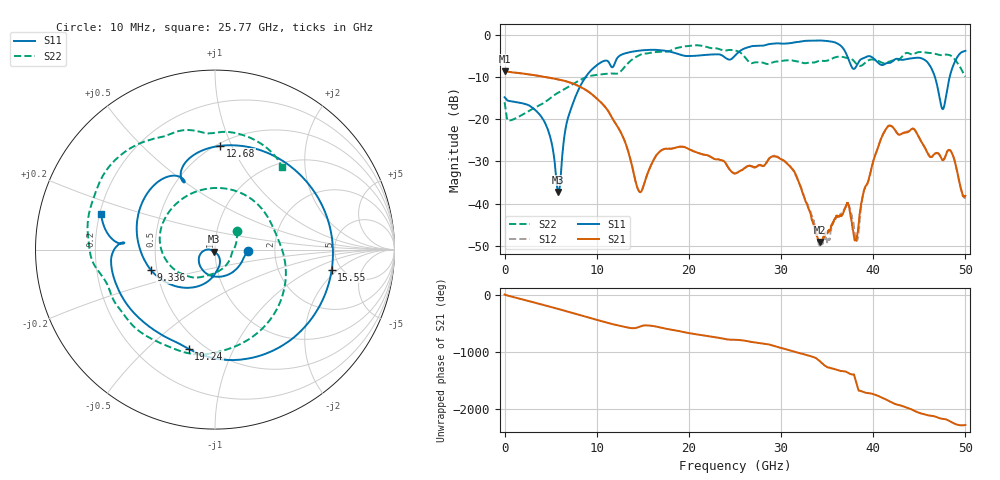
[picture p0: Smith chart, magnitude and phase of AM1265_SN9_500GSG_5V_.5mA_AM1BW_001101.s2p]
!Keysight Technologies,N5245B,MY58422270,A.16.20.02
!Date: Thursday, March 05, 2026 00:44:23
!Correction: S11(C  2-Port  )
!S21(C  2-Port  )
!S12(C  2-Port  )
!S22(C  2-Port  )
!S2P File: Measurements: S11, S21, S12, S22:
# Hz S  dB  R 50
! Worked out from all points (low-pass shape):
!   3201 points, 10 MHz to 50 GHz, reference 50 ohm
!   highest |S21| = -8.66 dB at 10 MHz (marker M1); lowest = -49.0 dB at 34.25 GHz (marker M2)
!   |S21| within 3 dB of the highest: start of sweep to 7.536 GHz
!   lowest |S11| = -37.2 dB at 5.837 GHz (marker M3), VSWR 1.03, Z = 49.2 - j1.12 ohm
!   |S11| at or under -10 dB: start of sweep to 8.809 GHz; 46.69 GHz to 48.29 GHz (1.601 GHz wide, 3.37 % of centre)
!   |S22| runs from -20.4 to -2.5 dB; largest |S21 - S12| = 0.0083
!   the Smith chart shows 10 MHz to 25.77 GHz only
!   S11 on the Smith chart (normalised r, x): 10 MHz: 1.44, -0.02; 9.336 GHz: 0.46, -0.12; 12.68 GHz: 0.52, +0.91; 15.55 GHz: 4.19, -1.66; 19.24 GHz: 0.42, -0.68; 25.77 GHz: 0.21, +0.15
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1e7  -14.81 -1.9  -8.66 2.9  -8.64 1.9  -15.98 40.9
2.040844e9  -16.30 -80.8  -9.21 -86.8  -9.21 -86.8  -18.81 -69.6
4.165419e9  -19.96 -152.9  -9.91 -176.8  -9.90 -176.8  -16.26 -108.6
5.836959e9  -37.20 -124.4  -10.58 110.4  -10.57 110.5  -13.70 -132.7
8.352081e9  -11.61 -125.8  -12.49 -4.4  -12.48 -4.3  -10.55 -178.4
9.336259e9  -8.54 -162.2  -13.85 -49.8  -13.84 -49.7  -9.75 154.2
1.267934e10  -4.75 87.1  -23.39 169.4  -23.38 169.4  -8.52 -0.6
1.455397e10  -3.80 21.9  -36.88 153.2  -36.87 153.0  -4.95 -85.9
1.555377e10  -3.61 -9.7  -32.62 -177.4  -32.71 -177.1  -4.42 -118.5
1.667854e10  -3.62 -43.1  -27.97 154.5  -27.93 154.8  -4.10 -145.0
1.924053e10  -4.85 -104.8  -26.49 73.1  -26.51 73.1  -2.89 171.8
2.5005e10  -4.96 174.9  -32.85 -68.4  -32.81 -69.2  -3.74 70.3
2.577047e10  -3.54 162.5  -32.00 -77.9  -32.08 -78.9  -4.55 51.2
3.031644e10  -2.12 83.7  -29.78 135.0  -29.89 135.8  -6.14 -43.6
3.334708e10  -1.40 35.7  -43.80 -1.9  -42.85 -1.7  -6.61 -133.3
3.425315e10  -1.38 19.9  -49.04 -89.8  -49.30 -88.1  -6.17 -153.2
3.717444e10  -5.01 -40.9  -39.78 83.4  -40.44 83.4  -5.51 150.1
3.825235e10  -7.12 -22.1  -47.66 -141.8  -48.53 20.5  -7.07 133.9
4.167354e10  -6.71 -54.0  -21.57 -57.7  -21.52 -57.8  -6.42 110.2
4.515722e10  -5.54 -102.0  -25.09 84.1  -25.06 84.5  -4.11 73.4
4.770358e10  -16.85 69.3  -29.39 -13.2  -29.41 -12.9  -4.77 41.7
5e10  -3.83 -71.7  -38.14 -118.9  -38.52 -128.6  -9.91 8.8
